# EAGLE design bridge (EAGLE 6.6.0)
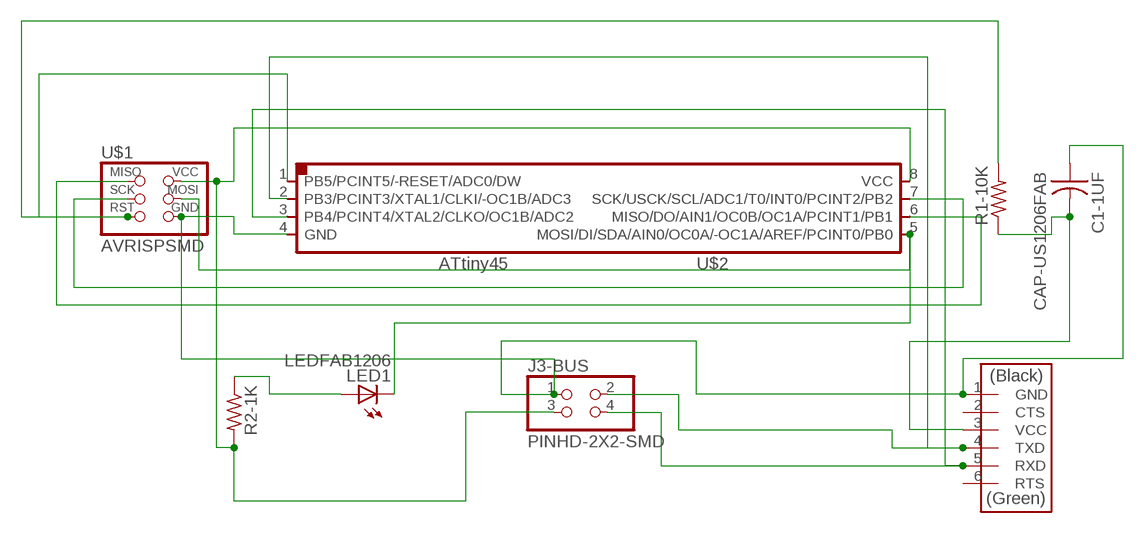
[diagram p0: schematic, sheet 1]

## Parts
C1-1UF  CAP-US1206FAB  [C1206FAB]
J3-BUS  PINHD-2X2-SMD  [2X02SMD]
LED1  LEDFAB1206  [LED1206FAB]
R1-10K  RES-US1206FAB  [R1206FAB]
R2-1K  RES-US1206FAB  [R1206FAB]
U$1  AVRISPSMD  [2X03SMD]
U$2  ATTINY45SI  [SOIC8]
U$5  FTDI-SMD-HEADER  [1X06SMD]

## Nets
N$1: C1-1UF.1 J3-BUS.1 U$1.6(GND) U$2.4(GND) U$5.1(GND)
N$2: J3-BUS.4 U$2.3(PB4/PCINT4/XTAL2/CLKO/OC1B/ADC2) U$5.5(RXD)
N$3: J3-BUS.2 U$2.2(PB3/PCINT3/XTAL1/CLKI/-OC1B/ADC3) U$5.4(TXD)
N$4: J3-BUS.3 R2-1K.2 U$1.2(VCC) U$2.8(VCC)
N$5: U$1.3(SCK) U$2.7(SCK/USCK/SCL/ADC1/T0/INT0/PCINT2/PB2)
N$6: U$1.1(MISO) U$2.6(MISO/DO/AIN1/OC0B/OC1A/PCINT1/PB1)
N$7: R1-10K.2 U$1.5(RST) U$2.1(PB5/PCINT5/-RESET/ADC0/DW)
N$8: LED1.2(C) U$1.4(MOSI) U$2.5(MOSI/DI/SDA/AIN0/OC0A/-OC1A/AREF/PCINT0/PB0)
N$9: LED1.1(A) R2-1K.1
N$10: C1-1UF.2 R1-10K.1 U$5.3(VCC)
Unconnected: U$5.2(CTS) U$5.6(RTS)

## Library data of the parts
C1-1UF = fab:CAP-US
J3-BUS = fab:PINHD-2X2-SMD
LED1 = fab:LED: LED
R1-10K R2-1K = fab:RES-US: Resistor (US Symbol)
U$1 = fab:AVRISP
U$2 = fab:ATTINY45
U$5 = fab:FTDI-SMD-HEADER

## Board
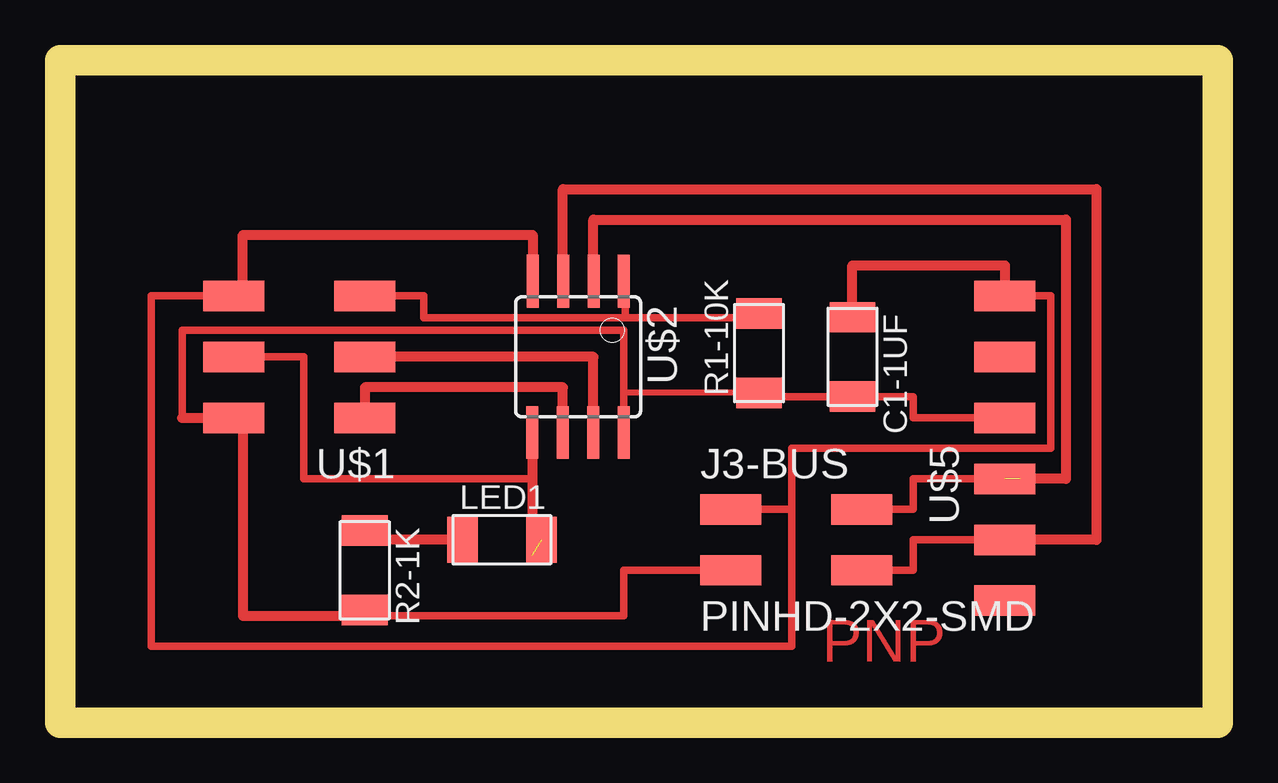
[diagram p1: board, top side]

Size 48.24 x 27.61 mm. Coordinates in mm from the lower left corner, seen from the top.
Outline: 0,0 48.24,0 48.24,27.61 0,27.61 0,0
Copper layers (1*16): Top 0.035mm / dielectric 1.5mm / Bottom 0.035mm
Design rules "default": minimum track width 10mil, minimum drill 24mil, track to track 8mil, track to pad 8mil, pad to pad 8mil, via to via 8mil, smd to smd 8mil, copper to edge 40mil, drill to drill 8mil, minimum pad ring 10mil, minimum via ring 8mil, stop-mask expansion 4mil, vias tented up to drill 0mil, thermal gap 10mil

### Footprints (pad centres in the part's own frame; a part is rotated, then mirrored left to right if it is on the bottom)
C1206FAB = smd 1.27 x 1.905: 1 -1.651,0; 2 1.651,0
2X02SMD = smd 2.54 x 1.27: 1 -2.54,1.27; 2 2.92,1.27; 3 -2.54,-1.27; 4 2.92,-1.27
LED1206FAB = smd 1.27 x 1.905: 1 -1.651,0; 2 1.651,0
R1206FAB = smd 1.27 x 1.905: 1 -1.651,0; 2 1.651,0
2X03SMD = smd 2.54 x 1.27: 1 -2.54,2.54; 2 2.92,2.54; 3 -2.54,0; 4 2.92,0; 5 -2.54,-2.54; 6 2.92,-2.54
SOIC8 = smd 0.5 x 2.2: 1 -1.905,-3.154; 2 -0.645,-3.154; 3 0.625,-3.154; 4 1.895,-3.154; 5 1.905,3.154; 6 0.635,3.154; 7 -0.635,3.154; 8 -1.905,3.154
1X06SMD = smd 2.54 x 1.27: 1 0,6.35; 2 0,3.81; 3 0,1.27; 4 0,-1.27; 5 0,-3.81; 6 0,-6.35

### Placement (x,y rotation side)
C1-1UF  33.02,15.24 270 top
J3-BUS  30.48,7.62 0 top
LED1  18.41,7.62 0 top
R1-10K  29.12,15.39 90 top
R2-1K  12.7,6.35 270 top
U$1  10.16,15.24 180 top
U$2  21.59,15.24 180 top
U$5  39.37,11.43 0 top

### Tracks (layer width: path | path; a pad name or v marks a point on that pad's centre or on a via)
N$1
  Top 0.305: C1-1UF.1 33.02,16.51 | 30.48,8.89 30.48,11.43 41.27,11.43 41.27,17.78 U$5.1 | J3-BUS.1 30.48,8.89 | 30.48,8.89 30.48,3.17 3.81,3.17 3.81,17.78 U$1.6
  Top 0.406: 19.68,18.39 U$2.4 19.7,20.32 7.62,20.32 7.62,17.78 U$1.6 | C1-1UF.1 33.02,19.05 39.37,19.05 U$5.1
N$2
  Top 0.305: J3-BUS.4 35.56,6.35 35.56,7.62 U$5.5
  Top 0.406: U$2.3 20.95,22.23 43.18,22.23 43.18,7.62 U$5.5
N$3  (1 unrouted)
  Top 0.305: J3-BUS.2 35.56,8.89 35.56,10.16 U$5.4
  Top 0.406: U$2.2 22.23,20.95 41.91,20.95 41.91,10.16 40.01,10.16
N$4
  Top 0.305: J3-BUS.3 23.5,6.35 23.5,4.45 12.7,4.45 | 5.08,12.7 5.09,12.7 5.09,16.35 23.5,16.35 U$2.8
  Top 0.406: 5.08,12.7 U$1.2 7.62,12.7 7.62,4.45 12.7,4.45 R2-1K.2
N$5
  Top 0.406: U$2.7 22.23,15.24 U$1.3
N$6
  Top 0.406: U$2.6 20.95,13.97 12.7,13.97 U$1.1
N$7
  Top 0.305: U$1.5 15.15,17.78 15.15,16.87 23.54,16.87 | 23.54,16.87 29.12,16.87 R1-10K.2 | U$2.1 23.54,18.39 23.54,16.87
N$8  (1 unrouted)
  Top 0.305: U$1.4 10.16,15.24 10.16,10.16 19.68,10.16
  Top 0.406: U$2.5 19.68,10.16 19.68,6.99
N$9
  Top 0.406: LED1.1 12.7,7.62 R2-1K.1
N$10
  Top 0.254: 23.48,13.63 23.48,13.74 R1-10K.1 29.12,13.59
  Top 0.305: 29.12,13.59 C1-1UF.2 35.56,13.59 35.56,12.7 U$5.3

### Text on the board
Top: PNP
